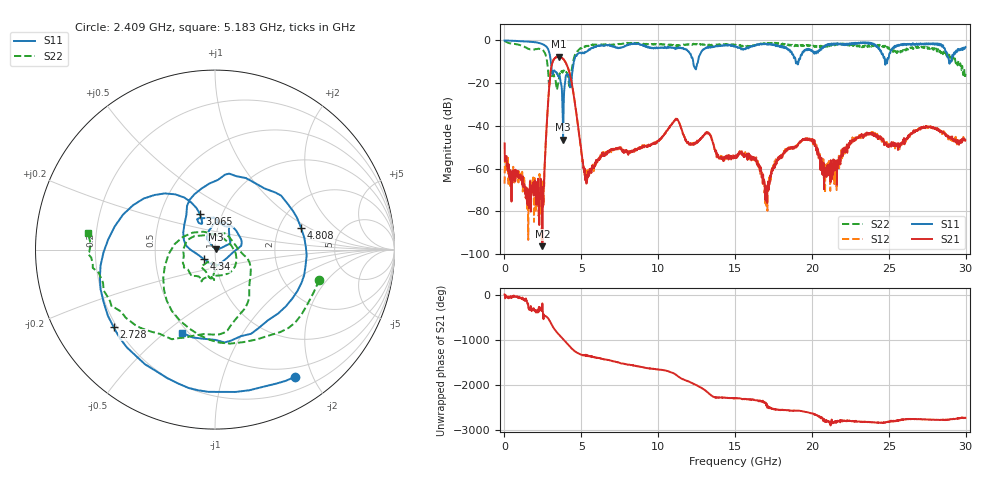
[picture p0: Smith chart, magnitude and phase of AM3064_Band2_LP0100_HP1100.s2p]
# Hz S DB R 50.0
!freq dBS11 angS11 dBS21 angS21 dBS12 angS12 dBS22 angS22
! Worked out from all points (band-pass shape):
!   1600 points, 10 MHz to 29.98 GHz, reference 50 ohm
!   highest |S21| = -7.65 dB at 3.534 GHz (marker M1); lowest = -96.3 dB at 2.465 GHz (marker M2)
!   |S21| within 3 dB of the highest: 3.108 GHz to 4 GHz (891.5 MHz wide, 25.1 % of centre)
!   lowest |S11| = -46.5 dB at 3.815 GHz (marker M3), VSWR 1.01, Z = 50.4 + j0.24 ohm
!   |S11| at or under -10 dB: 3.017 GHz to 4.514 GHz (1.496 GHz wide, 39.7 % of centre); 12.28 GHz to 12.59 GHz (310 MHz wide, 2.49 % of centre); 18.95 GHz to 19.12 GHz (176.5 MHz wide, 0.927 % of centre)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
!   |S22| runs from -23.2 to -0.2 dB; largest |S21 - S12| = 0.013
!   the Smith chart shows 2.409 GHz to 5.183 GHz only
!   S11 on the Smith chart (normalised r, x): 2.409 GHz: 0.37, -1.75; 2.728 GHz: 0.19, -0.33; 3.065 GHz: 0.78, +0.33; 4.34 GHz: 0.88, -0.09; 4.808 GHz: 2.65, +0.85; 5.183 GHz: 0.46, -0.57
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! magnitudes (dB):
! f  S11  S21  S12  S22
! 10 MHz  -0.1  -48.2  -67.1  -0.2
! 2.409 GHz  -1.5  -74.6  -67.7  -4.4
! 2.465 GHz  -1.8  -96.3  -65.3  -4.4
! 2.728 GHz  -3.0  -42.4  -42.2  -8.1
! 3.065 GHz  -13.3  -11.8  -11.8  -16.7
! 3.534 GHz  -17.0  -7.6  -7.8  -18.3
! 3.815 GHz  -46.5  -8.6  -8.6  -14.4
! 4.34 GHz  -21.8  -18.6  -18.5  -16.2
! 4.808 GHz  -6.1  -41.4  -41.2  -4.6
! 5.015 GHz  -6.2  -53.1  -53.1  -3.7
! 5.183 GHz  -6.0  -61.7  -61.9  -3.0
! 10 GHz  -3.5  -47.0  -47.1  -1.9
! 11.18 GHz  -3.5  -37.1  -36.9  -2.5
! 15 GHz  -2.7  -54.4  -54.9  -2.0
! 16.34 GHz  -2.3  -55.0  -55.0  -2.3
! 17.05 GHz  -1.9  -73.5  -70.7  -1.5
! 18.32 GHz  -3.2  -51.4  -51.2  -1.9
! 19.99 GHz  -4.7  -46.8  -47.1  -2.3
! 21.3 GHz  -1.9  -59.0  -61.3  -1.7
! 23.12 GHz  -1.4  -45.3  -45.0  -3.0
! 25 GHz  -8.1  -49.9  -49.8  -3.3
! 29.98 GHz  -3.2  -46.7  -46.8  -15.7
